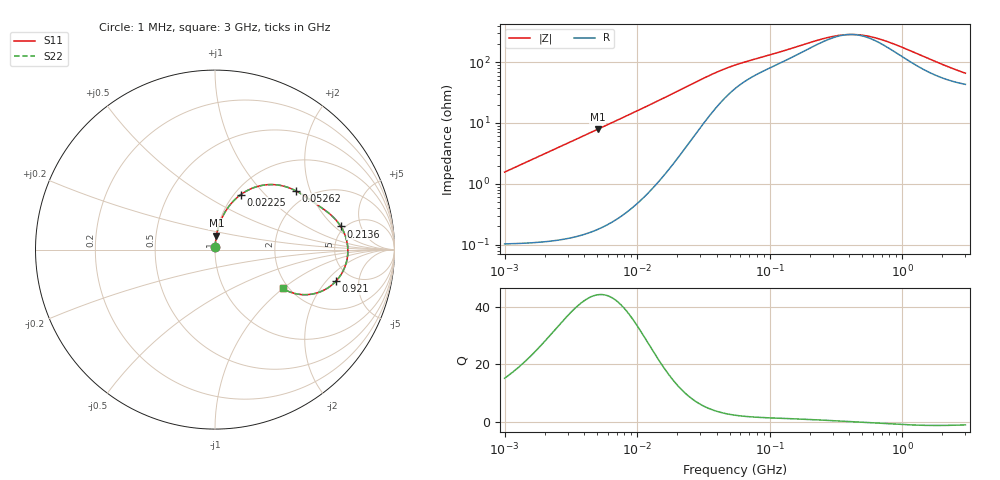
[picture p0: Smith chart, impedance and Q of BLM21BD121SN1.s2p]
! BLM21BD121SN1
# Hz S RI R 50
!Freq.(Hz) S11(Real) S11(Imag) S21(Real) S21(Imag) S12(Real) S12(Imag) S22(Real) S22(Imag)
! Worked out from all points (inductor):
!   401 points, 1 MHz to 3 GHz, reference 50 ohm
!   read as one part in series: L = 248 nH near 1.041 MHz
!   highest Q = 44.2 at 5.06 MHz (marker M1), where L = 249 nH
!   self-resonance near 406.8 MHz
!   S11 on the Smith chart (normalised r, x): 1 MHz: 1.00, +0.03; 22.25 MHz: 1.07, +0.74; 52.62 MHz: 1.68, +1.60; 213.6 MHz: 4.63, +2.43; 921 MHz: 3.76, -2.56; 3 GHz: 1.86, -0.99
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1000000  0.00127 0.0155  0.9987 -0.0155  0.9987 -0.0155  0.00127 0.0155
3823119  0.00496 0.0592  0.995 -0.0592  0.995 -0.0592  0.00496 0.0592
5059610  0.00796 0.0783  0.992 -0.0783  0.992 -0.0783  0.00796 0.0783
8861669  0.0227 0.136  0.9773 -0.136  0.9773 -0.136  0.0227 0.136
1.461624e7  0.0617 0.2182  0.9383 -0.2182  0.9383 -0.2182  0.0617 0.2182
2.225279e7  0.1425 0.3055  0.8575 -0.3055  0.8575 -0.3055  0.1425 0.3055
2.829425e7  0.22 0.3466  0.78 -0.3466  0.78 -0.3466  0.22 0.3466
3.456417e7  0.2983 0.362  0.7017 -0.362  0.7017 -0.362  0.2983 0.362
5.262293e7  0.4495 0.3281  0.5505 -0.3281  0.5505 -0.3281  0.4495 0.3281
5.477226e7  0.4607 0.3221  0.5393 -0.3221  0.5393 -0.3221  0.4607 0.3221
9.034013e7  0.5653 0.2529  0.4347 -0.2529  0.4347 -0.2529  0.5653 0.2529
2.094008e8  0.6983 0.1329  0.3017 -0.1329  0.3017 -0.1329  0.6983 0.1329
2.136344e8  0.7007 0.1293  0.2993 -0.1293  0.2993 -0.1293  0.7007 0.1293
3.124888e8  0.7326 0.0551  0.2674 -0.0551  0.2674 -0.0551  0.7326 0.0551
4.219165e8  0.7403 -0.00781  0.2597 0.00781  0.2597 0.00781  0.7403 -0.00781
5.583748e8  0.7325 -0.0686  0.2675 0.0686  0.2675 0.0686  0.7325 -0.0686
8.005644e8  0.6972 -0.1468  0.3028 0.1468  0.3028 0.1468  0.6972 -0.1468
9.209708e8  0.6745 -0.1753  0.3255 0.1753  0.3255 0.1753  0.6745 -0.1753
1.268618e9  0.6027 -0.2281  0.3973 0.2281  0.3973 0.2281  0.6027 -0.2281
1.645649e9  0.5301 -0.2495  0.4699 0.2495  0.4699 0.2495  0.5301 -0.2495
2.134733e9  0.4565 -0.2472  0.5435 0.2472  0.5435 0.2472  0.4565 -0.2472
3e9  0.3766 -0.2166  0.6234 0.2166  0.6234 0.2166  0.3766 -0.2166
